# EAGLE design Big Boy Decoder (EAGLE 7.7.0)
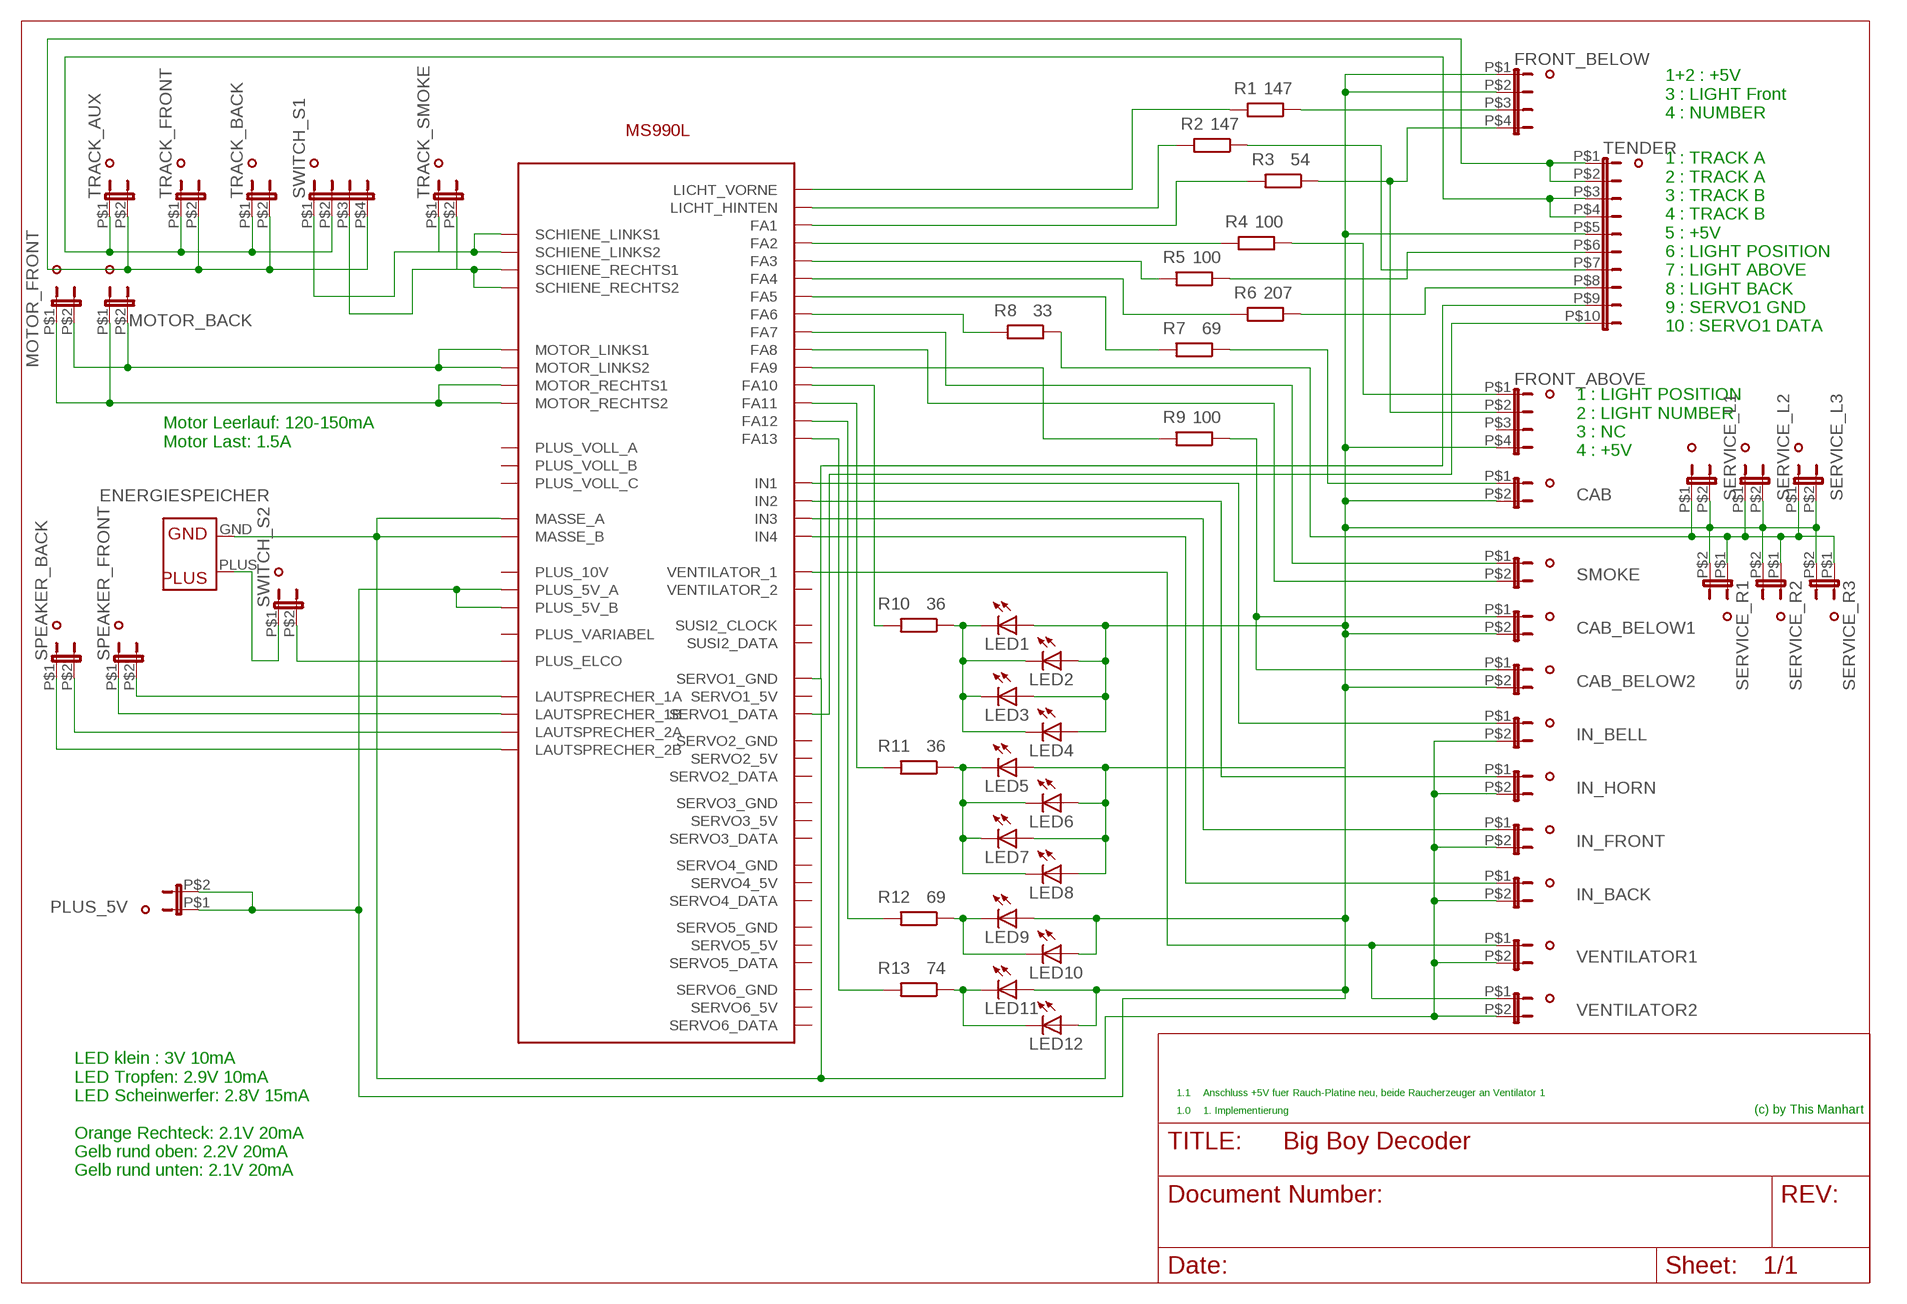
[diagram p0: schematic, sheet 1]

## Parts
CAB  DUBOX_2POL  [DUBOX_2POL_STIFTLEISTE]
CAB_BELOW1  DUBOX_2POL  [DUBOX_2POL_STIFTLEISTE]
CAB_BELOW2  DUBOX_2POL  [DUBOX_2POL_STIFTLEISTE]
FRONT_ABOVE  DUBOX_4POLNORMAL  [DUBOX_4POL_STIFTLEISTE_1R]
FRONT_BELOW  DUBOX_4POL2REIHIG  [DUBOX_4POL_STIFTLEISTE_2R]
IN_BACK  DUBOX_2POL  [DUBOX_2POL_STIFTLEISTE]
IN_BELL  DUBOX_2POL  [DUBOX_2POL_STIFTLEISTE]
IN_FRONT  DUBOX_2POL  [DUBOX_2POL_STIFTLEISTE]
IN_HORN  DUBOX_2POL  [DUBOX_2POL_STIFTLEISTE]
LED1  LED  [LED3MM_OHNE]
LED2  LED  [LED3MM_OHNE]
LED3  LED  [LED3MM_OHNE]
LED4  LED  [LED3MM_OHNE]
LED5  LED  [LED3MM_OHNE]
LED6  LED  [LED3MM_OHNE]
LED7  LED  [LED3MM_OHNE]
LED8  LED  [LED3MM_OHNE]
LED9  LED  [LED3MM_OHNE]
LED10  LED  [LED3MM_OHNE]
LED11  LED  [LED3MM_OHNE]
LED12  LED  [LED3MM_OHNE]
MOTOR_BACK  DUBOX_2POL  [DUBOX_2POL_STIFTLEISTE]
MOTOR_FRONT  DUBOX_2POL  [DUBOX_2POL_STIFTLEISTE]
PLUS_5V  DUBOX_2POL  [DUBOX_2POL_STIFTLEISTE]
R1  147  R-EU_R0805  [R0805]
R2  147  R-EU_R0805  [R0805]
R3  54  R-EU_R0805  [R0805]
R4  100  R-EU_R0805  [R0805]
R5  100  R-EU_R0805  [R0805]
R6  207  R-EU_R0805  [R0805]
R7  69  R-EU_R0805  [R0805]
R8  33  R-EU_R0805  [R0805]
R9  100  R-EU_R0805  [R0805]
R10  36  R-EU_R0805  [R0805]
R11  36  R-EU_R0805  [R0805]
R12  69  R-EU_R0805  [R0805]
R13  74  R-EU_R0805  [R0805]
SERVICE_L1  DUBOX_2POL  [DUBOX_2POL_STIFTLEISTE]
SERVICE_L2  DUBOX_2POL  [DUBOX_2POL_STIFTLEISTE]
SERVICE_L3  DUBOX_2POL  [DUBOX_2POL_STIFTLEISTE]
SERVICE_R1  DUBOX_2POL  [DUBOX_2POL_STIFTLEISTE]
SERVICE_R2  DUBOX_2POL  [DUBOX_2POL_STIFTLEISTE]
SERVICE_R3  DUBOX_2POL  [DUBOX_2POL_STIFTLEISTE]
SMOKE  DUBOX_2POL  [DUBOX_2POL_STIFTLEISTE]
SPEAKER_BACK  DUBOX_2POL  [DUBOX_2POL_STIFTLEISTE]
SPEAKER_FRONT  DUBOX_2POL  [DUBOX_2POL_STIFTLEISTE]
SWITCH_S1  DUBOX_4POL2REIHIG  [DUBOX_4POL_STIFTLEISTE_2R]
SWITCH_S2  DUBOX_2POL  [DUBOX_2POL_STIFTLEISTE]
TENDER  DUBOX_10POL2R  [DUBOX_10POL_STIFTLEISTE_2R]
TRACK_AUX  DUBOX_2POL  [DUBOX_2POL_STIFTLEISTE]
TRACK_BACK  DUBOX_2POL  [DUBOX_2POL_STIFTLEISTE]
TRACK_FRONT  DUBOX_2POL  [DUBOX_2POL_STIFTLEISTE]
TRACK_SMOKE  DUBOX_2POL  [DUBOX_2POL_STIFTLEISTE]
U$1  MS990L  [MS990L]
U$2  ENERGIESPEICHER  [ENERGIESPEICHER]
VENTILATOR1  DUBOX_2POL  [DUBOX_2POL_STIFTLEISTE]
VENTILATOR2  DUBOX_2POL  [DUBOX_2POL_STIFTLEISTE]

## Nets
N$1: SWITCH_S1.P$1 TRACK_SMOKE.P$1 U$1.15(SCHIENE_LINKS1) U$1.16(SCHIENE_LINKS2)
N$2: SWITCH_S1.P$3 TRACK_SMOKE.P$2 U$1.17(SCHIENE_RECHTS1) U$1.18(SCHIENE_RECHTS2)
N$3: SWITCH_S1.P$4 TENDER.P$1 TENDER.P$2 TRACK_AUX.P$2 TRACK_BACK.P$2 TRACK_FRONT.P$2
N$4: SWITCH_S1.P$2 TENDER.P$3 TENDER.P$4 TRACK_AUX.P$1 TRACK_BACK.P$1 TRACK_FRONT.P$1
N$5: MOTOR_BACK.P$1 MOTOR_FRONT.P$1 U$1.19(MOTOR_RECHTS1) U$1.28(MOTOR_RECHTS2)
N$6: MOTOR_BACK.P$2 MOTOR_FRONT.P$2 U$1.23(MOTOR_LINKS1) U$1.25(MOTOR_LINKS2)
N$7: SPEAKER_BACK.P$1 U$1.39(LAUTSPRECHER_2B)
N$8: SPEAKER_FRONT.P$1 U$1.27(LAUTSPRECHER_1B)
N$9: SPEAKER_BACK.P$2 U$1.40(LAUTSPRECHER_2A)
N$10: SPEAKER_FRONT.P$2 U$1.26(LAUTSPRECHER_1A)
N$11: SWITCH_S2.P$1 U$2.PLUS
N$13: FRONT_BELOW.P$3 R1.1
N$14: R1.2 U$1.3(LICHT_VORNE)
N$15: R12.2 U$1.31(FA12)
N$16: R2.2 U$1.2(LICHT_HINTEN)
N$17: FRONT_ABOVE.P$2 FRONT_BELOW.P$4 R3.1
N$18: R3.2 U$1.5(FA1)
N$19: R5.2 U$1.7(FA3)
N$20: R4.2 U$1.6(FA2)
N$21: R5.1 TENDER.P$6
N$22: R6.2 U$1.9(FA4)
N$23: R6.1 TENDER.P$8
N$24: R2.1 TENDER.P$7
N$25: FRONT_ABOVE.P$1 R4.1
N$26: R7.2 U$1.10(FA5)
N$27: CAB.P$1 R7.1
N$28: R8.2 U$1.12(FA6)
N$29: R8.1 SERVICE_L1.P$1 SERVICE_L2.P$1 SERVICE_L3.P$1 SERVICE_R1.P$1 SERVICE_R2.P$1 SERVICE_R3.P$1
N$30: SMOKE.P$1 U$1.36(FA7)
N$31: SMOKE.P$2 U$1.35(FA8)
N$32: R9.2 U$1.34(FA9)
N$33: CAB_BELOW1.P$1 CAB_BELOW2.P$1 R9.1
N$35: IN_BELL.P$1 U$1.4(IN1)
N$36: IN_HORN.P$1 U$1.8(IN2)
N$37: IN_FRONT.P$1 U$1.24(IN3)
N$38: IN_BACK.P$1 U$1.11(IN4)
N$40: U$1.41(VENTILATOR_1) VENTILATOR1.P$1 VENTILATOR2.P$1
N$41: R10.2 U$1.33(FA10)
N$42: LED1.K(C) LED2.K(C) LED3.K(C) LED4.K(C) R10.1
N$43: LED9.K(C) LED10.K(C) R12.1
N$44: R11.2 U$1.32(FA11)
N$45: LED5.K(C) LED6.K(C) LED7.K(C) LED8.K(C) R11.1
N$46: CAB.P$2 CAB_BELOW1.P$2 CAB_BELOW2.P$2 FRONT_ABOVE.P$4 FRONT_BELOW.P$1 FRONT_BELOW.P$2 LED1.A LED2.A LED3.A LED4.A LED5.A LED6.A LED7.A LED8.A LED9.A LED10.A LED11.A LED12.A PLUS_5V.P$1 PLUS_5V.P$2 SERVICE_L1.P$2 SERVICE_L2.P$2 SERVICE_L3.P$2 SERVICE_R1.P$2 SERVICE_R2.P$2 SERVICE_R3.P$2 TENDER.P$5 U$1.37(PLUS_5V_B) U$1.61(PLUS_5V_A)
N$47: SWITCH_S2.P$2 U$1.63(PLUS_ELCO)
N$48: R13.2 U$1.29(FA13)
N$49: LED11.K(C) LED12.K(C) R13.1
N$50: IN_BACK.P$2 IN_BELL.P$2 IN_FRONT.P$2 IN_HORN.P$2 TENDER.P$9 U$1.22(MASSE_A) U$1.60(SERVO1_GND) U$1.62(MASSE_B) U$2.GND VENTILATOR1.P$2 VENTILATOR2.P$2
N$51: TENDER.P$10 U$1.58(SERVO1_DATA)
Unconnected: FRONT_ABOVE.P$3 U$1.1(SUSI2_DATA) U$1.13(PLUS_VOLL_A) U$1.14(SUSI2_CLOCK) U$1.20(PLUS_VOLL_B) U$1.21(PLUS_VOLL_C) U$1.30(PLUS_VARIABEL) U$1.38(PLUS_10V) U$1.42(VENTILATOR_2) U$1.43(SERVO6_DATA) U$1.44(SERVO6_5V) U$1.45(SERVO6_GND) U$1.46(SERVO5_DATA) U$1.47(SERVO5_5V) U$1.48(SERVO5_GND) U$1.49(SERVO4_DATA) U$1.50(SERVO4_5V) U$1.51(SERVO4_GND) U$1.52(SERVO3_DATA) U$1.53(SERVO3_5V) U$1.54(SERVO3_GND) U$1.55(SERVO2_DATA) U$1.56(SERVO2_5V) U$1.57(SERVO2_GND) U$1.59(SERVO1_5V)

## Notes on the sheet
- 1+2 : +5V
  3 : LIGHT Front
  4 : NUMBER
- 1 : TRACK A
  2 : TRACK A
  3 : TRACK B
  4 : TRACK B
  5 : +5V
  6 : LIGHT POSITION
  7 : LIGHT ABOVE
  8 : LIGHT BACK
  9 : SERVO1 GND
  10 : SERVO1 DATA
- Motor Leerlauf: 120-150mA
  Motor Last: 1.5A
- 1 : LIGHT POSITION
  2 : LIGHT NUMBER
  3 : NC
  4 : +5V
- IN_HORN
- 1.1 | Anschluss +5V fuer Rauch-Platine neu, beide Raucherzeuger an Ventilator 1
- 1.0 | 1. Implementierung | (c) by This Manhart
- LED klein : 3V 10mA
  LED Tropfen: 2.9V 10mA
  LED Scheinwerfer: 2.8V 15mA
  
  Orange Rechteck: 2.1V 20mA
  Gelb rund oben: 2.2V 20mA
  Gelb rund unten: 2.1V 20mA

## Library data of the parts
CAB CAB_BELOW1 CAB_BELOW2 IN_BACK IN_BELL IN_FRONT IN_HORN MOTOR_BACK MOTOR_FRONT PLUS_5V SERVICE_L1-SERVICE_L3 SERVICE_R1-SERVICE_R3 SMOKE SPEAKER_BACK SPEAKER_FRONT SWITCH_S2 TRACK_AUX TRACK_BACK TRACK_FRONT TRACK_SMOKE VENTILATOR1 VENTILATOR2 = 0_mm:DUBOX_2POL: DUBOX 2pol Buchse
FRONT_ABOVE FRONT_BELOW SWITCH_S1 = 0_mm:DUBOX_4POL
LED1-LED12 = 0_mm:LED: LED
R1-R13 = resistor:R-EU_: RESISTOR, European symbol
TENDER = 0_mm:DUBOX_10POL
U$1 = 0_digital:MS990L
U$2 = 0_mm:ENERGIESPEICHER

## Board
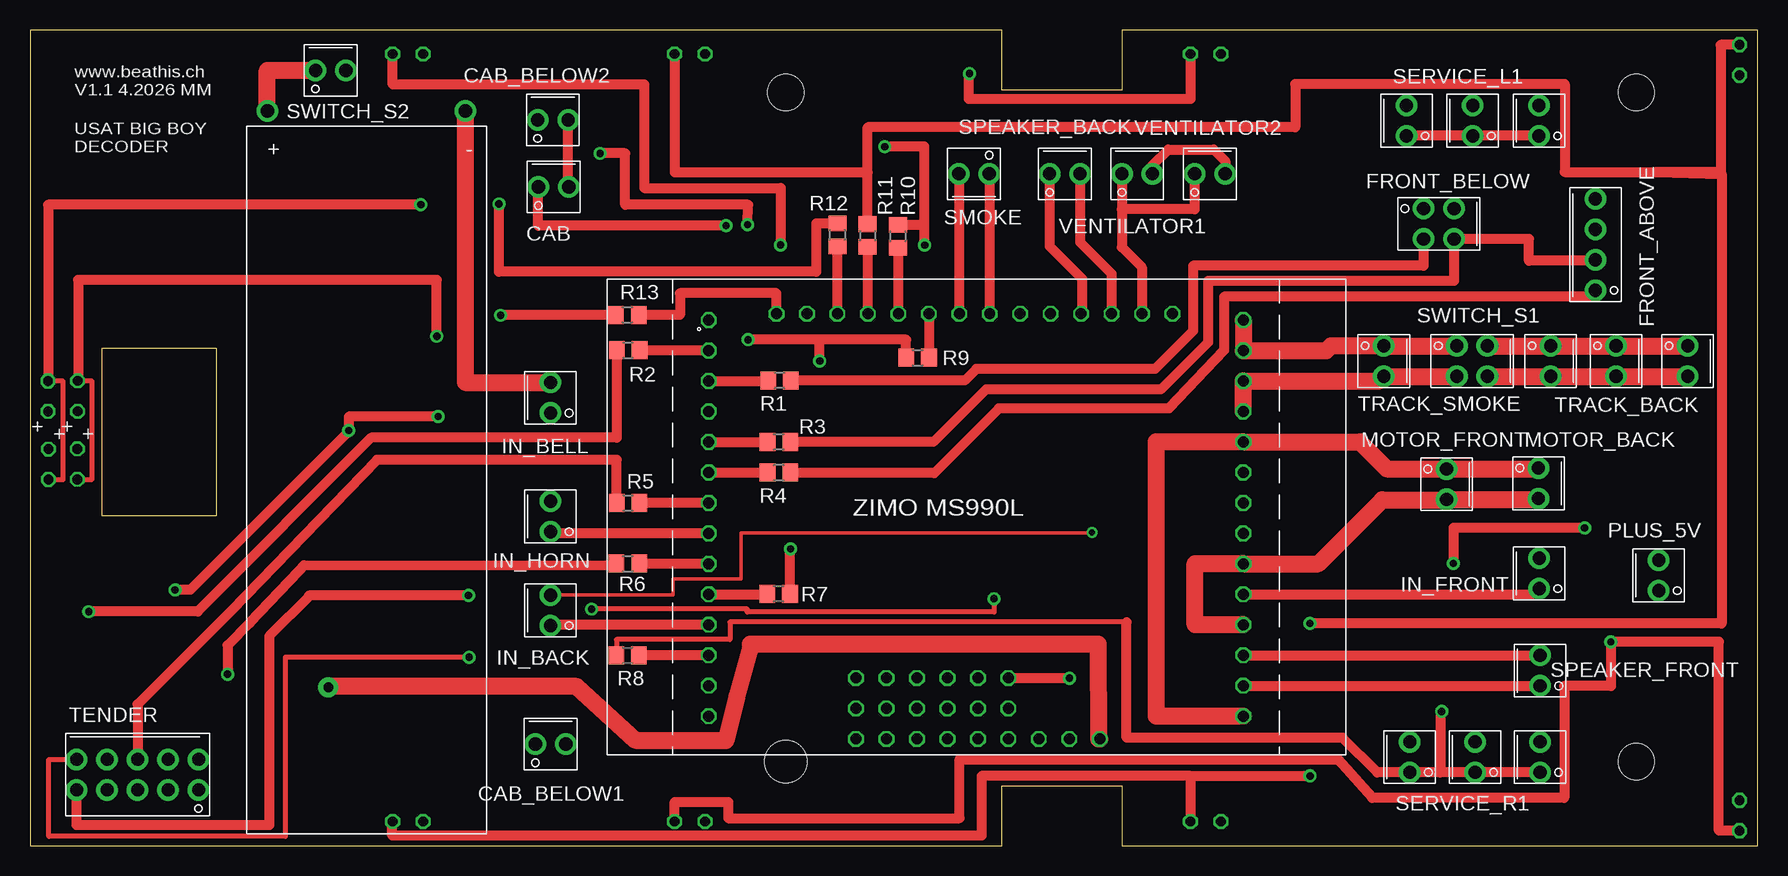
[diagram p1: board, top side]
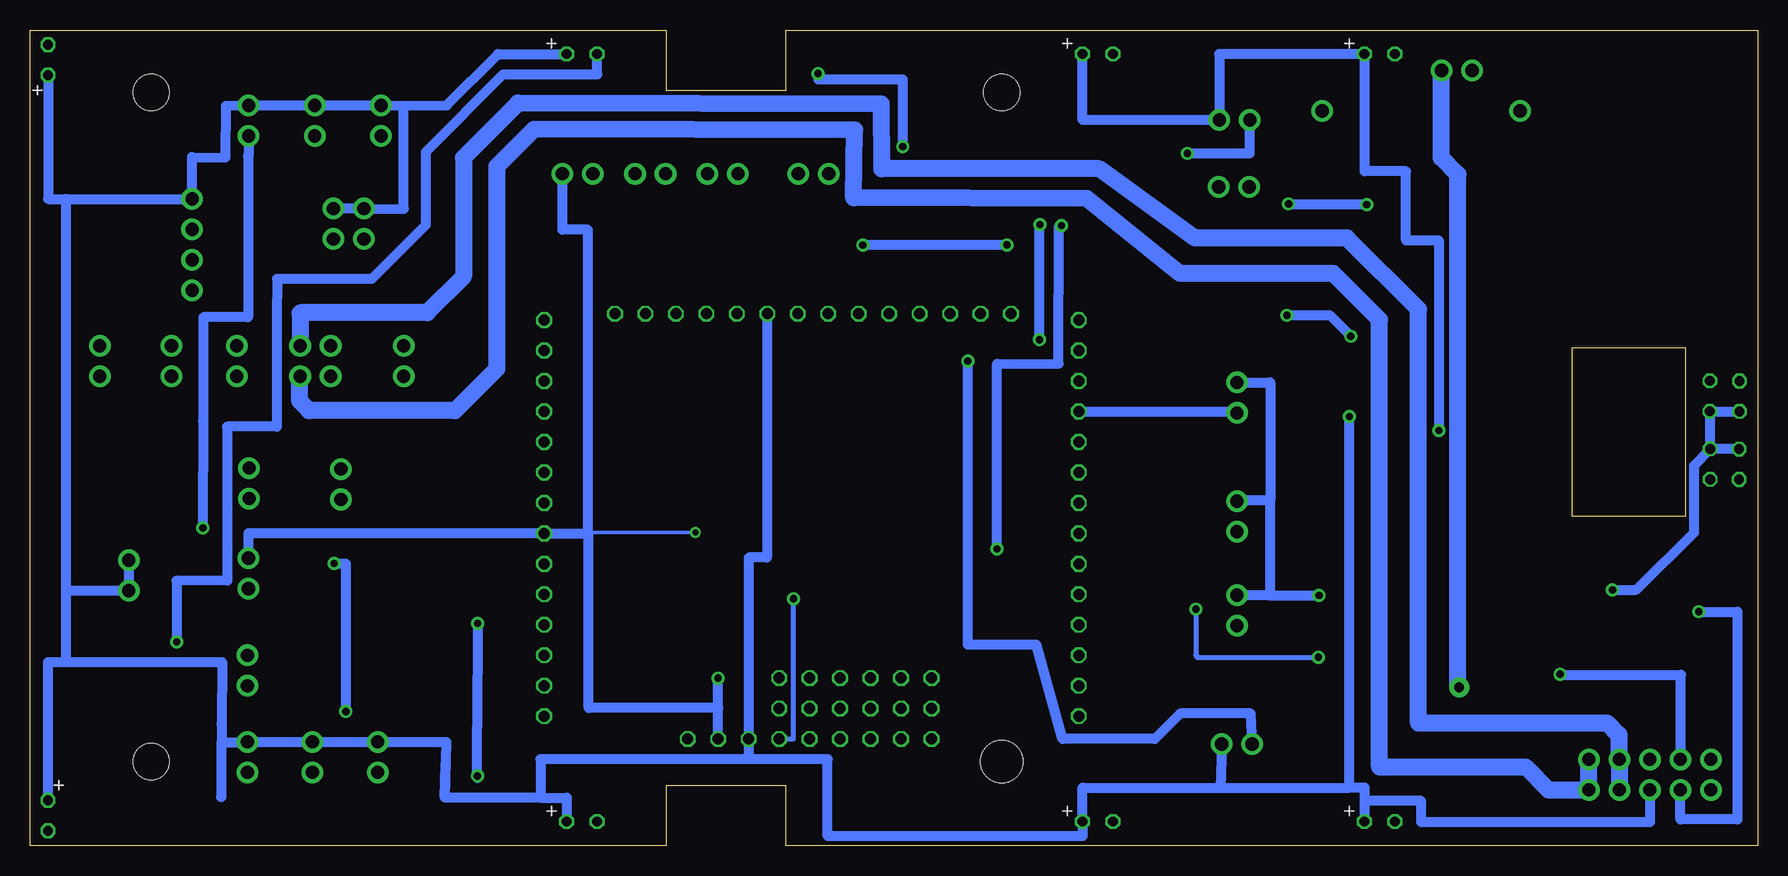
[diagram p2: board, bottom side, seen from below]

Size 144 x 68 mm. Coordinates in mm from the lower left corner, seen from the top.
Outline: 144,0 144,68 91,68 91,63 81,63 81,68 0,68 0,0 81,0 81,5 91,5 91,0 144,0
Outline: 6,41.5 15.5,41.5 15.5,27.5 6,27.5 6,41.5
Copper layers (1*16): Top 0.035mm / dielectric 1.5mm / Bottom 0.035mm
Design rules "PCB-POOL Standard": minimum track width 0.15mm, minimum drill 0.3mm, track to track 0.15mm, track to pad 0.15mm, pad to pad 0.15mm, via to via 0.15mm, smd to smd 0.15mm, copper to edge 0.3mm, drill to drill 0.2mm, minimum pad ring 0.2mm, minimum via ring 0.15mm, stop-mask expansion 0.075mm, vias tented up to drill 0mil, thermal gap 0.2mm
Holes 3 mm at 63,62.8 133.9,7 133.9,62.8
Holes 3.5 mm at 63,7

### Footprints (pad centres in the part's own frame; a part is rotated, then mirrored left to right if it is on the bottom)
DUBOX_2POL_STIFTLEISTE = drill 1.1 pad 1.8: P$1 -1.27,0; P$2 1.27,0
DUBOX_4POL_STIFTLEISTE_1R = drill 1.1 pad 1.8: P$1 -1.27,0; P$2 1.27,0; P$3 3.81,0; P$4 6.35,0
DUBOX_4POL_STIFTLEISTE_2R = drill 1.1 pad 1.8: P$1 -1.27,0; P$2 -1.27,2.54; P$3 1.27,0; P$4 1.27,2.54
LED3MM_OHNE = drill 0.813 octagon: A -1.27,0; K 1.27,0
R0805 = smd 1.3 x 1.5: 1 -0.95,0; 2 0.95,0
DUBOX_10POL_STIFTLEISTE_2R = drill 1.1 pad 1.8: P$1 8.89,0; P$2 8.89,2.54; P$3 6.35,0; P$4 6.35,2.54; P$5 3.81,0; P$6 3.81,2.54; P$7 1.27,0; P$8 1.27,2.54; P$9 -1.27,0; P$10 -1.27,2.54
MS990L = drill 0.914 octagon: 1 0,0; 2 0,-2.54; 3 0,-5.08; 4 0,-7.62; 5 0,-10.16; 6 0,-12.7; 7 0,-15.24; 8 0,-17.78; 9 0,-20.32; 10 0,-22.86; 11 0,-25.4; 12 0,-27.94; 13 0,-30.48; 14 0,-33.02; 15 44.56,0; 16 44.56,-2.54; 17 44.56,-5.08; 18 44.56,-7.62; 19 44.56,-10.16; 20 44.56,-12.7; 21 44.56,-15.24; 22 44.56,-17.78; 23 44.56,-20.32; 24 44.56,-22.86; 25 44.56,-25.4; 26 44.56,-27.94; 27 44.56,-30.48; 28 44.56,-33.02; 29 5.64,0.53; 30 8.18,0.53; 31 10.72,0.53; 32 13.26,0.53; 33 15.8,0.53; 34 18.34,0.53; 35 20.88,0.53; 36 23.42,0.53; 37 25.96,0.53; 38 28.5,0.53; 39 31.04,0.53; 40 33.58,0.53; 41 36.12,0.53; 42 38.66,0.53; 43 12.27,-34.93; 44 12.27,-32.39; 45 12.27,-29.85; 46 14.81,-34.93; 47 14.81,-32.39; 48 14.81,-29.85; 49 17.35,-34.93; 50 17.35,-32.39; 51 17.35,-29.85; 52 19.89,-34.93; 53 19.89,-32.39; 54 19.89,-29.85; 55 22.43,-34.93; 56 22.43,-32.39; 57 22.43,-29.85; 58 24.97,-34.93; 59 24.97,-32.39; 60 24.97,-29.85; 61 27.51,-34.93; 62 30.05,-34.93; 63 32.59,-34.93
ENERGIESPEICHER = drill 1.1 pad 1.8: GND 16.5,0; PLUS 0,0

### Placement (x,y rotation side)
CAB  43.64,54.91 0 top
CAB_BELOW1  43.39,8.45 0 top
CAB_BELOW2  43.59,60.5 0 top
FRONT_ABOVE  130.49,47.56 90 top
FRONT_BELOW  116.16,51.84 270 top
IN_BACK  43.39,19.61 90 top
IN_BELL  43.39,37.34 90 top
IN_FRONT  125.8,22.68 90 top
IN_HORN  43.39,27.43 90 top
LED1  31.5,66 0 bottom
LED2  55,2 0 bottom
LED3  98,66 0 bottom
LED4  142.5,2.5 270 bottom
LED5  31.5,2 0 bottom
LED6  55,66 0 bottom
LED7  98,2 0 bottom
LED8  142.5,65.5 90 bottom
LED9  1.5,37.46 90 top
LED10  1.54,31.79 270 top
LED11  3.97,37.47 90 top
LED12  3.94,31.8 270 top
MOTOR_BACK  125.74,30.2 270 top
MOTOR_FRONT  118.08,30.12 270 top
PLUS_5V  135.76,22.52 90 top
R1  62.48,38.78 180 top
R2  49.86,41.3 0 top
R3  62.43,33.64 180 top
R4  62.43,31.09 180 top
R5  49.85,28.57 0 top
R6  49.83,23.51 0 top
R7  62.4,20.98 180 top
R8  49.81,15.86 0 top
R9  73.99,40.67 0 top
R10  72.34,50.79 270 top
R11  69.82,50.86 270 top
R12  67.3,50.91 270 top
R13  49.79,44.25 0 top
SERVICE_L1  114.74,60.44 90 top
SERVICE_L2  120.26,60.44 90 top
SERVICE_L3  125.78,60.44 90 top
SERVICE_R1  115.01,7.37 90 top
SERVICE_R2  120.45,7.37 90 top
SERVICE_R3  125.87,7.37 90 top
SMOKE  78.69,56.01 180 top
SPEAKER_BACK  86.26,56.01 0 top
SPEAKER_FRONT  125.88,14.59 90 top
SWITCH_S1  118.94,40.39 270 top
SWITCH_S2  25.07,64.63 0 top
TENDER  5.16,4.64 0 top
TRACK_AUX  138.18,40.39 270 top
TRACK_BACK  126.76,40.39 270 top
TRACK_FRONT  132.21,40.39 270 top
TRACK_SMOKE  112.85,40.39 270 top
U$1  56.58,43.81 0 top
U$2  19.79,61.25 0 top
VENTILATOR1  92.29,56.01 0 top
VENTILATOR2  98.35,56.01 0 top

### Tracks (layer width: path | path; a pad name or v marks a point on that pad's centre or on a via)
N$1
  Top 1.422: U$1.15 U$1.16 108.05,41.27 108.46,41.68 112.83,41.68 TRACK_SMOKE.P$1 SWITCH_S1.P$1
N$2
  Top 1.422: U$1.18 U$1.17 112.46,38.73 TRACK_SMOKE.P$2 SWITCH_S1.P$3
N$3
  Top 1.422: SWITCH_S1.P$4 TRACK_BACK.P$2 TRACK_FRONT.P$2 TRACK_AUX.P$2
  Bottom 1.422: SWITCH_S1.P$4 121.52,39.08 121.52,37.06 120.73,36.27 108.57,36.27 105.09,39.75 105.09,56.62 102,59.71 75.26,59.66 75.34,54.01 55.9,53.95 48.13,47.69 35.36,47.69 31.51,43.84 31.51,6.55 19.33,6.55 17.42,4.64 TENDER.P$1 TENDER.P$2
N$4
  Top 1.422: SWITCH_S1.P$2 TRACK_BACK.P$1 TRACK_FRONT.P$1 TRACK_AUX.P$1
  Bottom 1.422: SWITCH_S1.P$2 121.49,44.39 121.45,44.43 110.89,44.43 107.87,47.45 107.87,57.35 103.32,61.9 73.03,61.83 72.99,56.42 54.87,56.42 46.88,50.65 34.21,50.65 28.27,44.71 28.27,10.21 12.54,10.21 11.56,9.23 11.56,7.23 TENDER.P$4 TENDER.P$3
N$5
  Top 1.422: MOTOR_BACK.P$1 125.66,31.39 MOTOR_FRONT.P$1 118.06,31.41 113.1,31.41 110.86,33.65 U$1.19 93.86,33.65 93.86,10.8 U$1.28
N$6
  Top 1.422: MOTOR_BACK.P$2 125.66,28.85 MOTOR_FRONT.P$2 118.06,28.83 112.72,28.83 107.38,23.49 U$1.23 101.14,23.51 97.12,23.51 97.12,18.41 U$1.25
N$7
  Top 0.813: SPEAKER_BACK.P$1 84.99,49.97 87.7,47.26 87.7,44.42 U$1.39
N$8
  Top 0.813: U$1.27 SPEAKER_FRONT.P$1
N$9
  Top 0.813: SPEAKER_BACK.P$2 87.53,50.31 90.16,47.68 U$1.40
N$10
  Top 0.813: U$1.26 SPEAKER_FRONT.P$2
N$11
  Top 1.422: U$2.PLUS 19.79,64.63 SWITCH_S2.P$1
N$13
  Top 0.813: FRONT_BELOW.P$3 116.16,48.34 96.94,48.34 96.94,42.9 93.78,39.74 78.89,39.74 77.93,38.78 R1.1
N$14
  Top 0.813: U$1.3 61.53,38.73 R1.2
N$15
  Top 0.813: U$1.31 R12.2
N$16
  Top 0.813: U$1.2 50.84,41.27 R2.2
N$17
  Top 0.813: R3.1 75.31,33.65 79.69,38.03 94.27,38.03 98.19,41.95 98.19,47.07 118.7,47.07 FRONT_BELOW.P$4 124.95,50.57 124.95,48.77 130.49,48.77 FRONT_ABOVE.P$2
N$18
  Top 0.813: U$1.5 R3.2
N$19
  Top 0.813: U$1.7 R5.2
N$20
  Top 0.813: U$1.6 61.48,31.11 R4.2
N$21
  Top 0.813: R5.1 48.9,32.15 28.93,32.15 16.73,19.54 8.97,11.78 TENDER.P$6
N$22
  Top 0.813: U$1.9 50.8,23.49 R6.2
N$23  (via drill 0.6 pad 1.02)
  Top 0.813: R6.1 48.88,23.33 22.84,23.36 22.42,22.88 18.33,18.56 16.46,16.69 v16.46,14.29
  Bottom 0.813: v16.46,14.29 16.42,14.25 6.39,14.25 6.43,14.21 TENDER.P$8
N$24  (via drill 0.6 pad 1.02)
  Top 0.813: R2.1 48.91,34.01 28.45,34.01 13.98,19.51 v4.9,19.51 v4.9,19.5
  Bottom 0.813: v4.9,19.5 1.68,19.5 1.68,2.18 6.43,2.18 TENDER.P$7
N$25
  Top 0.813: FRONT_ABOVE.P$1 130.49,45.77 99.53,45.77 99.53,41.28 94.94,36.44 80.77,36.44 75.39,31.06 63.41,31.06 R4.1
N$26
  Top 0.813: U$1.10 61.42,20.95 R7.2
N$27  (via drill 0.6 pad 1.02)
  Top 0.813: R7.1 63.35,24.69 v63.39,24.73 | v58.02,51.68 42.37,51.68 CAB.P$1
  Bottom 0.813: v63.39,24.73 63.39,40.15 58.27,40.17 58.24,51.63 v58.02,51.68
N$28
  Top 0.813: U$1.12 R8.2
N$29  (via drill 0.6 pad 1.02)
  Top 0.406: 91.41,18.63 58.34,18.63 58.34,17.17 48.88,17.17 48.88,15.86 R8.1
  Top 0.813: SERVICE_R3.P$1 SERVICE_R2.P$1 117.55,6.1 | 117.55,6.1 SERVICE_R1.P$1 112.3,6.1 109.4,9 91.41,9 91.41,18.63 | SERVICE_L3.P$1 SERVICE_L2.P$1 SERVICE_L1.P$1 | v129.59,26.49 118.65,26.49 v118.65,23.51 | v117.67,11.17 117.55,11.17 117.55,6.1
  Bottom 0.813: 129.56,35.4 129.56,44.06 125.83,44.06 125.83,57.52 125.78,57.52 SERVICE_L3.P$1 | 129.56,35.4 129.59,35.4 | 129.56,35.4 129.59,26.98 v129.59,26.49 | v118.65,23.51 117.67,23.51 v117.67,11.17
N$30
  Top 0.813: SMOKE.P$1 79.96,44.38 U$1.36
N$31
  Top 0.813: SMOKE.P$2 77.42,44.38 U$1.35
N$32
  Top 0.813: U$1.34 74.92,40.67 R9.2
N$33  (via drill 0.6 pad 1.02)
  Top 0.813: R9.1 73.04,42.17 65.83,42.17 | 65.83,42.17 v59.85,42.17 | v59.82,51.78 59.87,53.42 49.62,53.43 49.62,57.71 v47.52,57.71 | v65.83,40.4 65.83,42.17
  Bottom 0.813: v59.85,42.17 59.85,51.78 v59.82,51.78 | v47.52,57.71 42.32,57.71 CAB_BELOW2.P$1 | CAB_BELOW1.P$1 42.24,11.02 48.11,11.02 50.25,8.88 57.93,8.88 60.11,16.74 65.83,16.74 v65.83,40.4
N$35
  Bottom 0.813: U$1.4 43.51,36.19 IN_BELL.P$1
N$36
  Top 0.813: U$1.8 43.58,26.03 IN_HORN.P$1
N$37
  Top 0.813: U$1.24 125.8,20.95 IN_FRONT.P$1
N$38
  Top 0.813: U$1.11 43.51,18.41 IN_BACK.P$1
N$40
  Top 0.813: VENTILATOR1.P$1 91.02,53.06 | 91.02,53.06 91.02,49.88 92.68,48.22 92.68,44.36 U$1.41 | VENTILATOR2.P$1 97.08,53.06 91.02,53.06
N$41
  Top 0.813: U$1.33 72.38,49.8 R10.2
N$42  (via drill 0.6 pad 1.02)
  Top 0.813: v62.57,50.08 62.57,54.82 51.19,54.82 51.19,63.44 30.23,63.44 LED1.K | v74.58,50.06 74.55,50.06 74.55,51.75 | 74.55,51.75 R10.1 | 74.55,51.75 74.55,58.28 v71.25,58.28 | LED4.K 140.78,1.23 140.78,16.98 v131.78,16.98 v131.78,16.97 131.78,13.3 127.88,13.3 127.88,3.97 111.89,3.97 109.01,7.2 77.49,7.2 77.49,2.28 58.19,2.28 58.19,3.64 53.73,3.64 LED2.K | LED3.K 96.73,62.23 78.27,62.23 78.27,64.37 v78.31,64.37
  Bottom 0.813: v131.78,16.97 131.78,22.1 127.55,22.08 127.58,34.93 123.42,34.93 123.42,44.03 123.41,47.24 115.52,47.24 111.02,51.74 111.02,57.83 104.55,64.3 96.71,64.3 96.73,64.32 LED3.K | v62.57,50.08 74.58,50.08 v74.58,50.06 | v71.25,58.28 71.25,63.89 78.31,63.89 v78.31,64.37
N$43  (via drill 0.6 pad 1.02)
  Top 0.406: LED10.K 2.75,30.52 2.75,38.72 LED9.K
  Top 0.813: R12.1 65.53,51.86 65.53,47.84 39.09,47.84 v39.09,53.5 | v32.58,53.43 1.5,53.43 LED9.K
  Bottom 0.813: v39.09,53.5 32.58,53.5 v32.58,53.43
N$44
  Top 0.813: U$1.32 69.84,49.89 R11.2
N$45  (via drill 0.6 pad 1.02)
  Top 0.813: 96.73,5.8 79.33,5.8 79.33,0.82 30.2,0.82 30.2,2 LED5.K | R11.1 69.82,56.14 | 69.82,56.14 69.82,59.89 105.47,59.89 105.47,63.5 127.92,63.5 127.92,56.15 135.54,56.15 | 135.54,56.15 141,55.98 141,18.51 v106.69,18.51 | LED8.K 140.92,66.77 140.92,56.16 135.54,56.16 135.54,56.15 | LED6.K 53.73,56.14 69.82,56.14 | 96.73,5.8 LED7.K | 96.73,5.8 v106.7,5.8
  Bottom 0.813: v106.69,18.51 106.71,9.94 106.71,5.63 v106.7,5.8
N$46  (via drill 0.6 pad 1.02)
  Top 0.813: CAB.P$2 44.86,54.91 CAB_BELOW2.P$2 | v12.09,21.32 13.37,21.32 26.57,34.52 v26.57,34.6 26.57,35.76 v34.03,35.76
  Bottom 0.813: 44.89,8.45 CAB_BELOW1.P$2 44.78,4.82 | 84.09,7.2 77.52,7.2 77.52,0.78 56.27,0.78 LED2.A 56.27,4.82 44.78,4.82 | 84.23,8.88 U$1.61 | U$1.61 84.09,7.2 | 84.09,7.2 101.44,7.2 101.44,3.99 | 101.44,3.99 109.42,3.99 | 109.42,3.99 109.37,6.78 | 109.42,3.99 109.3,8.64 SERVICE_R1.P$2 SERVICE_R2.P$2 SERVICE_R3.P$2 125.87,8.62 128.04,8.62 | 112.84,61.68 SERVICE_L1.P$2 SERVICE_L2.P$2 SERVICE_L3.P$2 127.65,61.68 127.7,57.37 130.49,57.4 FRONT_ABOVE.P$4 141,53.91 | 112.84,61.68 109.27,61.71 104.98,66 LED3.A | FRONT_BELOW.P$2 118.79,53.11 118.79,53.15 116.16,53.15 FRONT_BELOW.P$1 112.84,53.08 112.84,61.68 | LED12.A 5.28,31.67 5.28,26.09 10.04,21.39 10.11,21.32 v12.09,21.32 | LED10.A LED12.A | LED9.A LED11.A 3.97,33.1 LED12.A | 128.08,4.06 128.04,4.06 128.04,8.62 | 141,15.3 127.99,15.3 128.03,10.18 127.98,10.13 128.04,10.13 128.04,8.62 | 141,15.3 141,21.25 | 141,53.91 141,21.5 141,21.25 | U$1.37 82.57,44.34 82.57,24.02 84.09,24.02 U$1.61 | v26.57,34.6 26.57,50.47 29.31,50.47 29.31,56.22 32.74,56.22 32.74,66 LED1.A 44.86,66 CAB_BELOW2.P$2 56.27,60.5 LED6.A | LED8.A 142.5,53.91 141,53.91 | LED4.A 142.5,15.3 141,15.3 | 32.77,3.72 32.77,4.82 34.03,4.82 | 32.77,3.72 LED5.A | 44.78,4.82 34.03,4.82 | 101.44,3.99 99.27,3.99 LED7.A | 34.03,4.82 v34.03,35.76 | TENDER.P$5 8.97,1.95 28.03,1.95 28.03,3.72 32.77,3.72 | PLUS_5V.P$2 PLUS_5V.P$1 141,21.25
N$47  (via drill 0.8 pad 1.68)
  Top 1.422: U$1.63 89.07,8.88 89.03,16.8 60.03,16.8 60.09,16.61 58.92,12.41 58.02,8.77 50.46,8.78 45.57,13.27 24.95,13.27 v24.87,13.19
  Bottom 1.422: v24.87,13.19 24.97,13.19 24.97,55.95 26.36,57.34 26.36,64.61 SWITCH_S2.P$2
N$48
  Top 0.813: U$1.29 62.22,46.06 54.18,46.06 54.18,44.25 R13.2
N$49  (via drill 0.6 pad 1.02)
  Top 0.406: LED12.K 5.18,30.53 5.18,38.72 3.97,38.72 LED11.K
  Top 0.813: R13.1 39.24,44.25 v39.24,44.21 | v33.91,42.46 33.91,47.15 4,47.15 4,38.74 LED11.K
  Bottom 0.813: v39.24,44.21 35.66,44.21 v33.91,42.46
N$50  (via drill 0.5, 0.6 pad 1.02)
  Top 0.305: IN_BACK.P$2 53.6,20.88 53.6,22.22 59.28,22.22 59.28,26.05 88.54,26.05 v88.54,26.1
  Top 0.813: VENTILATOR1.P$2 93.56,56.71 94.88,58.03 98.67,58.03 99.63,57.07 VENTILATOR2.P$2 | v86.64,13.95 U$1.60 | v36.55,20.85 23.25,20.85 23.25,20.76 19.95,17.46 19.95,1.7 3.89,1.7 TENDER.P$9
  Top 1.422: U$2.GND 36.29,38.61 IN_BELL.P$2
  Bottom 0.305: v88.54,26.1 97.43,26.1 97.43,26.03
  Bottom 0.813: IN_BELL.P$2 40.61,38.61 40.61,28.77 | 40.61,28.77 43.45,28.77 IN_HORN.P$2 | IN_BACK.P$2 40.61,20.88 | 40.61,20.88 40.61,28.77 | IN_FRONT.P$2 125.8,26.03 U$1.22 97.48,26.03 | 97.48,26.03 97.48,51.34 99.62,51.34 VENTILATOR2.P$2 | U$1.62 86.63,11.46 86.64,11.46 | 86.64,11.46 97.43,11.46 97.43,26.03 97.48,26.03 | 86.64,11.46 v86.64,13.95 | 40.61,20.88 40.61,20.85 v36.55,20.85
N$51  (via drill 0.6 pad 1.02)
  Top 0.406: v80.36,20.58 80.36,19.46 59.79,19.46 59.79,19.71 v46.82,19.71 | v36.6,15.7 21.29,15.7 21.29,0.77 1.57,0.77 1.57,7.18 TENDER.P$10
  Bottom 0.406: U$1.58 80.36,8.88 v80.36,20.58 | v46.82,19.71 46.82,15.87 46.76,15.87 46.76,15.69 v36.61,15.69 v36.6,15.7

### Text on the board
tNames: www.beathis.ch / V1.1 4.2026 MM | USAT BIG BOY / DECODER | ZIMO MS990L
